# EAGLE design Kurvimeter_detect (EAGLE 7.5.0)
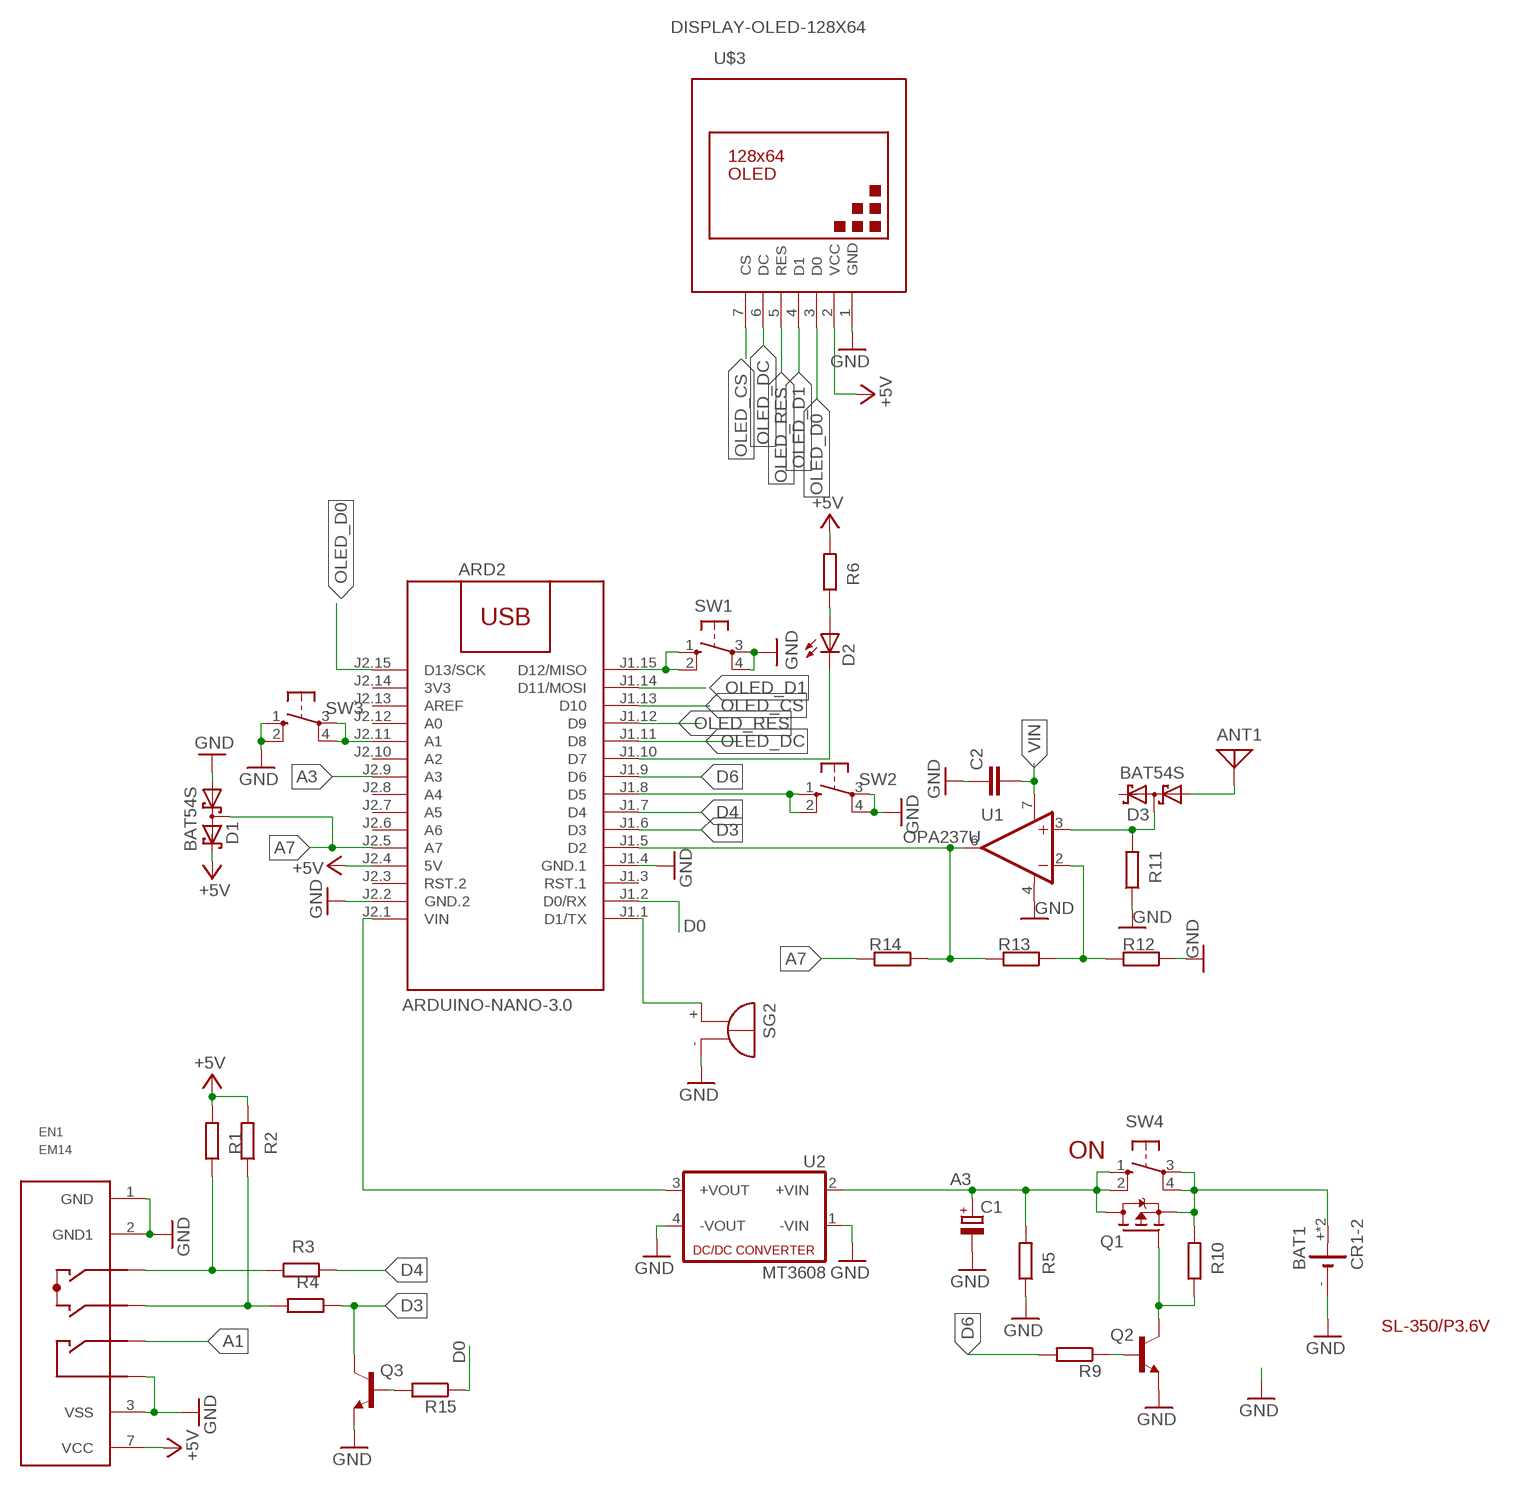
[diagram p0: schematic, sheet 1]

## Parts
ANT1  ANTENNA  [PAD-01]
ARD2  ARDUINO-NANO-3.0  [ARDUINO-NANO-3.0]
BAT1  CR1-2  [CR1-2]
C1  CPOL-EUSMCA  [SMC_A]
C2  C-EUC1206  [C1206]
D1  BAT54S  [SOT23]
D2  LED5MM  [LED5MM]
D3  BAT54S  [SOT23]
EN1  EM14  [EM14]
Q1  STR2P3LLH6  [SOT23]
Q2  BC817-16LT1SMD  [SOT23-BEC]
Q3  BC817-16LT1SMD  [SOT23-BEC]
R1  R-EU_R1206  [R1206]
R2  R-EU_R1206  [R1206]
R3  R-EU_R1206  [R1206]
R4  R-EU_R1206  [R1206]
R5  R-EU_R1206  [R1206]
R6  R-EU_R1206  [R1206]
R9  R-EU_R1206  [R1206]
R10  R-EU_R1206  [R1206]
R11  R-EU_R1206  [R1206]
R12  R-EU_R1206  [R1206]
R13  R-EU_R1206  [R1206]
R14  R-EU_R1206  [R1206]
R15  R-EU_R1206  [R1206]
SG2  BMT1205XH7.5  [BMT1205XH7.5]
SW1  10-XX  [B3F-10XX]
SW2  10-XX  [B3F-10XX]
SW3  10-XX  [B3F-10XX]
SW4  10-XX  [B3F-10XX]
U1  OPA237U  [SO08]
U2  MT3608  [MT3608]
U$3  DISPLAY-OLED-128X64  [DISPLAY-OLED-128X64]

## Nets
+5V: ARD2.J2.4(5V) D1.2(C2) EN1.7(VCC) R1.2 R2.2 R6.2 U$3.2(VCC)
A1: EN1.5(SW1)
A3: ARD2.J2.9(A3) C1.+ Q1.1(D) R5.2 SW4.1(S) SW4.2(S1) U2.2(+VIN)
A7: ARD2.J2.5(A7) D1.3(C1A2) R14.2
BAT: BAT1.+ BAT1.+@1(+) Q1.3(S) R10.2 SW4.3(P) SW4.4(P1)
D0: ARD2.J1.2(D0/RX) R15.1
D3: ARD2.J1.6(D3) Q3.C R4.1
D4: ARD2.J1.7(D4) R3.1
D6: ARD2.J1.9(D6) R9.2
GND: ARD2.J1.4(GND.1) ARD2.J2.2(GND.2) BAT1.- C1.- C2.1 D1.1(A1) EN1.1(GND) EN1.2(GND1) EN1.3(VSS) EN1.6(SW2) Q2.E Q3.E R5.1 R11.1 R12.1 SG2.- SW1.3(P) SW1.4(P1) SW2.3(P) SW2.4(P1) SW3.1(S) SW3.2(S1) U1.4(V-) U2.1(-VIN) U2.4(-VOUT) U$3.1(GND)
N$1: ARD2.J1.10(D7) D2.K(C)
N$2: ARD2.J1.8(D5) SW2.1(S) SW2.2(S1)
N$3: D3.3(C1A2) R11.2 U1.3(+IN)
N$4: D2.A R6.1
N$5: EN1.4(A) R1.1 R3.2
N$6: EN1.8(B) R2.1 R4.2
N$7: R12.2 R13.1 U1.2(-IN)
N$8: ARD2.J1.15(D12/MISO) SW1.1(S) SW1.2(S1)
N$9: ARD2.J1.5(D2) R13.2 R14.1 U1.6(OUT)
N$10: Q3.B R15.2
N$11: ANT1.1 D3.1(A1)
N$12: ARD2.J2.1(VIN) U2.3(+VOUT)
N$13: ARD2.J1.1(D1/TX) SG2.+
N$14: ARD2.J2.11(A1) SW3.3(P) SW3.4(P1)
N$16: Q1.2(G) Q2.C R10.1
N$18: Q2.B R9.1
OLED_CS: ARD2.J1.13(D10) U$3.7(CS)
OLED_D0: ARD2.J2.15(D13/SCK) U$3.3(D0)
OLED_D1: ARD2.J1.14(D11/MOSI) U$3.4(D1)
OLED_DC: ARD2.J1.11(D8) U$3.6(DC)
OLED_RES: ARD2.J1.12(D9) U$3.5(RES)
VIN: C2.2 U1.7(V+)
Unconnected: ARD2.J1.3(RST.1) ARD2.J2.3(RST.2) ARD2.J2.6(A6) ARD2.J2.7(A5) ARD2.J2.8(A4) ARD2.J2.10(A2) ARD2.J2.12(A0) ARD2.J2.13(AREF) D3.2(C2)

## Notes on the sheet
- ON
- SL-350/P3.6V

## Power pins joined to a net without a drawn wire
3V3: ARD2.J2.14(3V3)

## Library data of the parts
ANT1 = discrete:ANTENNA: Antenna
ARD2 = diy-modules:ARDUINO-NANO-3.0: Arduino Nano 3.0 and compatible devices More details available here: https://www.arduino.cc/en/Main/ArduinoBoardNano Click here to find device on ebay.com
BAT1 = battery:CR1-2
C1 = rcl:CPOL-EU: POLARIZED CAPACITOR, European symbol
C2 = rcl:C-EU: CAPACITOR, European symbol
D1 D3 = diode:BAT54S: Schottky Diodes Pin connection corrected 2011-05-04 Source: Fairchild .. BAT54.pdf
D2 = led:LED: LED
EN1 = switch-alps:EM14: 14 mm Rotary Optical Encoder w/Switch
Q1 = transistor-fet:STR2P3LLH6
Q2 Q3 = transistor-npn:BC817*: NPN Transistor
R1-R6 R9-R15 = rcl:R-EU_: RESISTOR, European symbol
SG2 = buzzer:BMT1205XH7.5: MAGNETIC TRANSDUCER; OC_FARNELL: unknown; OC_NEWARK: unknown
SW1-SW4 = switch-omron:10-XX: OMRON SWITCH; MPN: B3F-1000; OC_FARNELL: 176432; OC_NEWARK: 36M3542
U1 = burr-brown:OPA237: Operational Amplifiers Single-Supply, MicroAmplifier(TM) Series; MF: TEXAS INSTRUMENT CONNECTORS; MPN: OPA237UA; OC_FARNELL: 1800507; OC_NEWARK: 04M4584
U2 = dc-dc-converter:MT3608: DC DC Up Converter
U$3 = diy-modules:DISPLAY-OLED-128X64: 128x64 Dot Matrix OLED Module based on SSD1306 chip Variant with SPI interface More details available here: http://www.instructables.com/id/How-to-use-OLED-display-arduino-module/ SSD1306 datasheet: https://cdn-shop.adafruit.com/datasheets/SSD1306.pdf Click here to find device on ebay.com Note: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

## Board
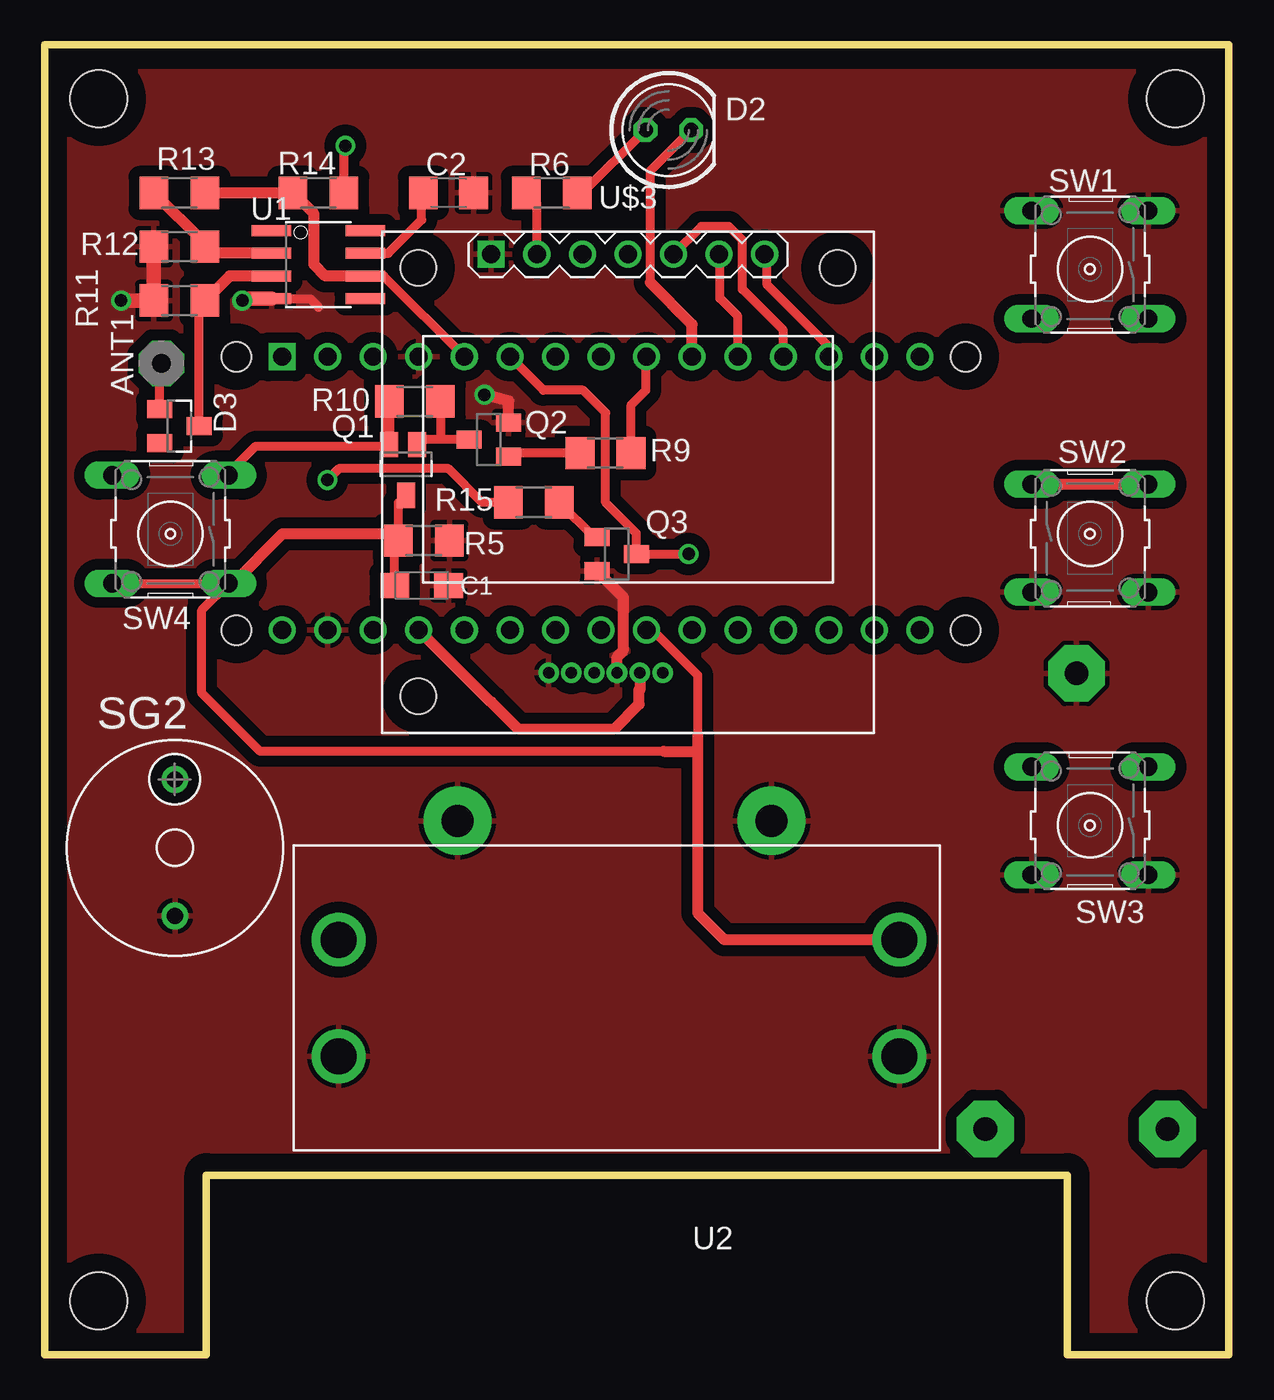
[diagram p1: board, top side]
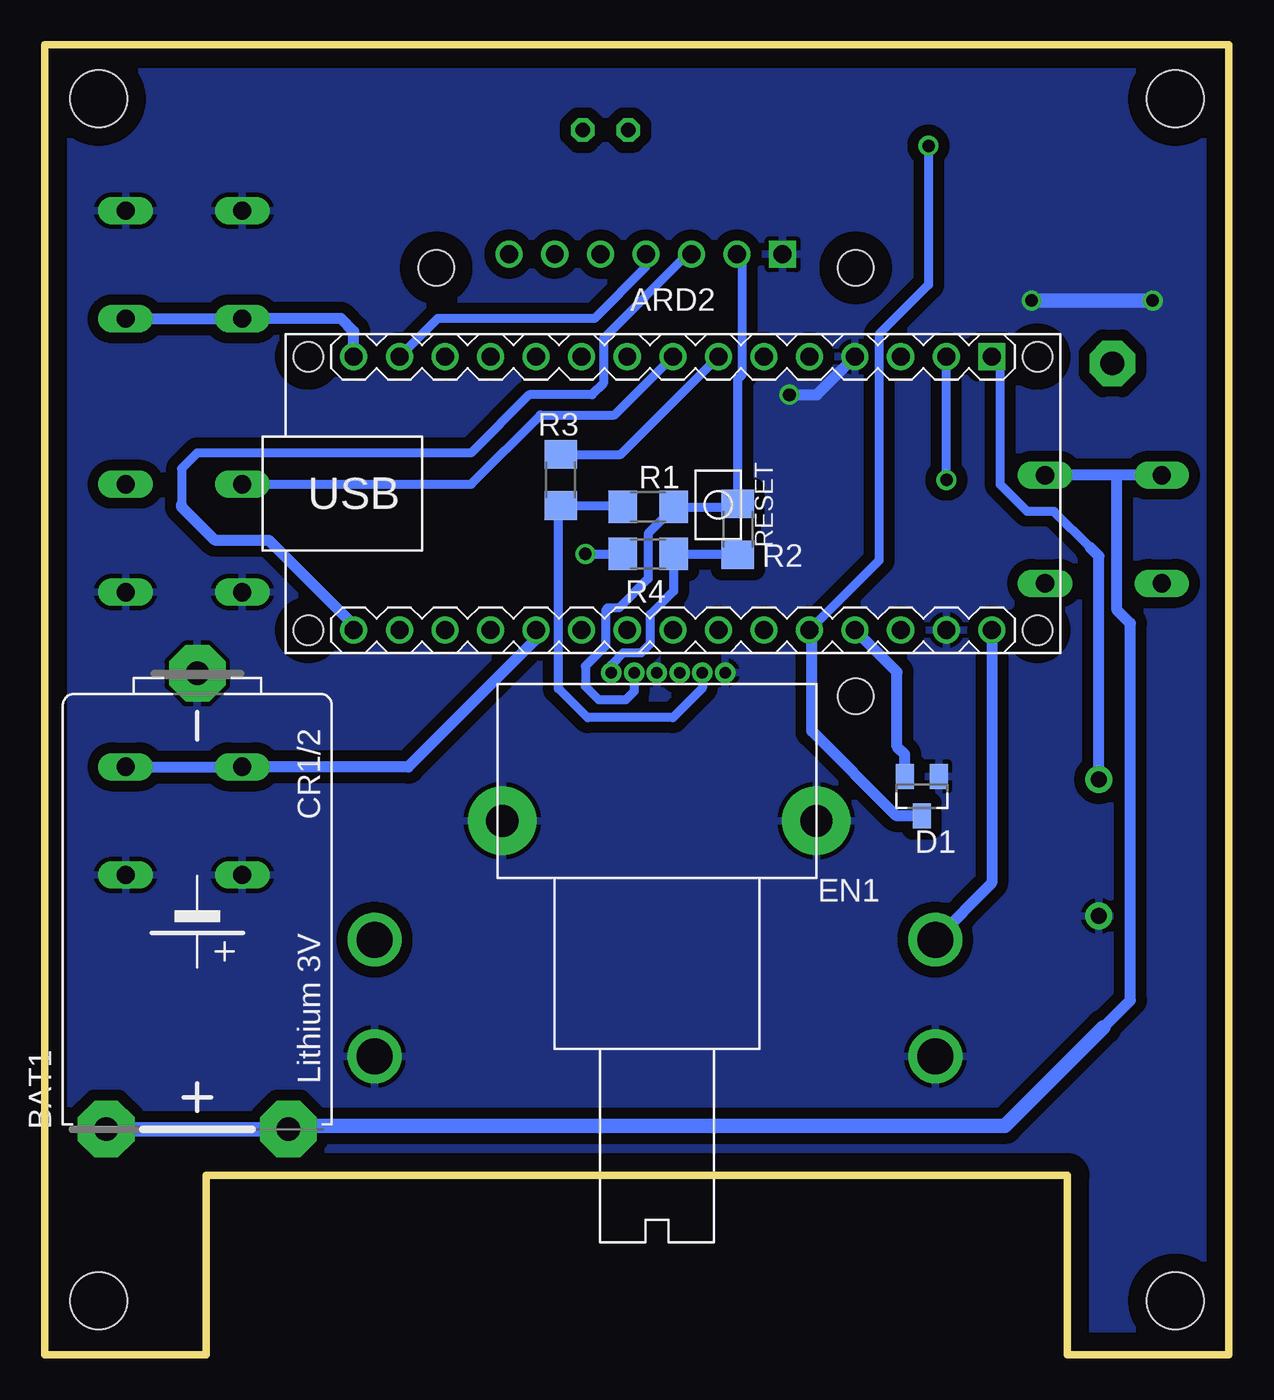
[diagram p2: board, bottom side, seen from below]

Size 66 x 73 mm. Coordinates in mm from the lower left corner, seen from the top.
Outline: 0,0 0,73 66,73 66,0 57,0 57,10 9,10 9,0 0,0
Copper layers (1*16): Top 0.035mm / dielectric 1.5mm / Bottom 0.035mm
Design rules "default *": minimum track width 10mil, minimum drill 15mil, track to track 6mil, track to pad 6mil, pad to pad 6mil, via to via 6mil, smd to smd 4mil, copper to edge 40mil, drill to drill 8mil, minimum pad ring 10mil, minimum via ring 8mil, stop-mask expansion 4mil, vias tented up to drill 0mil, thermal gap 10mil
Holes 3.2 mm at 3,70 63,70 3,3 63,3

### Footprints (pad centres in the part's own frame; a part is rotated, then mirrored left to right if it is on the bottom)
PAD-01 = drill 1.321 pad 2.54 octagon: 1 0,0
ARDUINO-NANO-3.0 = drill 1 square: J1.1 17.78,7.62 | drill 1: J1.2 15.24,7.62; J1.3 12.7,7.62; J1.4 10.16,7.62; J1.5 7.62,7.62; J1.6 5.08,7.62; J1.7 2.54,7.62; J1.8 0,7.62; J1.9 -2.54,7.62; J1.10 -5.08,7.62; J1.11 -7.62,7.62; J1.12 -10.16,7.62; J1.13 -12.7,7.62; J1.14 -15.24,7.62; J1.15 -17.78,7.62; J2.1 17.78,-7.62; J2.2 15.24,-7.62; J2.3 12.7,-7.62; J2.4 10.16,-7.62; J2.5 7.62,-7.62; J2.6 5.08,-7.62; J2.7 2.54,-7.62; J2.8 0,-7.62; J2.9 -2.54,-7.62; J2.10 -5.08,-7.62; J2.11 -7.62,-7.62; J2.12 -10.16,-7.62; J2.13 -12.7,-7.62; J2.14 -15.24,-7.62; J2.15 -17.78,-7.62 | hole 1.651: -20.32,7.62; -20.32,-7.62; 20.32,-7.62; 20.32,7.62
CR1-2 = drill 1.321 pad 3.15 octagon: + -11.43,-5.08; +@1 -11.43,5.08; - 13.97,0
SMC_A = smd 1.6 x 1.4: + -1.5,0; - 1.5,0
C1206 = smd 1.6 x 1.8: 1 -1.4,0; 2 1.4,0
SOT23 = smd 1 x 1.4: 1 -0.95,-1.1; 2 0.95,-1.1; 3 0,1.1
LED5MM = drill 0.813 octagon: A -1.27,0; K 1.27,0
EM14 = drill 1.8 pad 3.81: 1 0,0; 2 17.5,0 | drill 0.635 pad 0.889: 3 5.08,-8.255; 4 6.35,-8.255; 5 7.62,-8.255; 6 8.89,-8.255; 7 10.16,-8.255; 8 11.43,-8.255
SOT23' = smd 1 x 1.4: 1 0,1.735; 2 -0.632,-1.1; 3 0.95,-1.1
SOT23-BEC = smd 1 x 1.4: B -0.95,-1.1; C 0,1.1; E 0.95,-1.1
R1206 = smd 1.6 x 1.803: 1 -1.422,0; 2 1.422,0
BMT1205XH7.5 = drill 0.9 pad 1.5: + 3.8,0; - -3.8,0
B3F-10XX = drill 1.016 long: 1 -3.251,2.761; 2 3.251,2.761; 3 -3.251,-3.261; 4 3.251,-3.261
SO08 = smd 0.61 x 2.21: 1 -1.905,-2.616; 2 -0.635,-2.616; 3 0.635,-2.616; 4 1.905,-2.616; 5 1.905,2.616; 6 0.635,2.616; 7 -0.635,2.616; 8 -1.905,2.616
MT3608 = drill 2: 1 2.25,11.75; 2 2.25,5.25; 3 33.5,5.25; 4 33.5,11.75
DISPLAY-OLED-128X64 = drill 1 square: 1 -7.62,12.7 | drill 1: 2 -5.08,12.7; 3 -2.54,12.7; 4 0,12.7; 5 2.54,12.7; 6 5.08,12.7; 7 7.62,12.7 | hole 2: -11.684,11.938; 11.684,11.938; -11.684,-11.938

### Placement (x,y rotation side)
ANT1  6.5,55.25 0 top
ARD2  31,48 0 bottom
BAT1  57.5,24 90 bottom
C1  21,42.88 0 top
C2  22.5,64.75 180 top
D1  17.12,31.12 180 bottom
D2  34.75,68.25 0 top
D3  7.5,51.75 270 top
EN1  23,29.75 180 bottom
Q1  STR2P3LLH6  [SOT23']  20.12,49.62 180 top
Q2  24.75,51 90 top
Q3  31.88,44.62 270 top
R1  32.38,47.25 0 bottom
R2  27.38,46 90 bottom
R3  37.25,48.75 270 bottom
R4  32.38,44.62 0 bottom
R5  21.12,45.38 180 top
R6  28.25,64.75 180 top
R9  31.25,50.25 0 top
R10  20.62,53.12 180 top
R11  7.5,58.75 0 top
R12  7.5,61.75 0 top
R13  7.5,64.75 0 top
R14  15.25,64.75 0 top
R15  27.25,47.5 0 top
SG2  7.25,28.25 90 top
SW1  58.25,60.5 180 top
SW2  58.25,45.75 0 top
SW3  58.25,29.5 180 top
SW4  7,45.75 180 top
U1  15.25,60.75 270 top
U2  49.88,28.38 180 top
U$3  32.5,48.62 0 top

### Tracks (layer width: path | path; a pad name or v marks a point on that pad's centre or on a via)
+5V
  Top 0.5: U$3.2 27.42,64.16 R6.2
  Top 0.61: EN1.7 33.16,37.12 | 33.16,37.12 33.16,37.03 | ARD2.J2.4 24.84,36.38 24.88,36.38 26.38,34.88 31.75,34.88 33.12,36.25 33.12,37.09 33.16,37.12
  Bottom 0.5: U$3.2 27.12,61.03 27.12,54.62 27.38,54.38 R2.2 27.55,47.25 R1.2 30.95,47.17 32.38,45.75 32.38,43.25 34,41.62 34.62,41.62 34.75,41.5 34.75,39.5 35.88,38.38 35.88,37.25 35.12,36.5 33.62,36.5 33.16,36.97 EN1.7
  Bottom 0.61: D1.2 18.07,33.45 18.5,33.88 18.5,38.04 ARD2.J2.4
A3
  Top 0.5: C1.+ 19.5,45.17 R5.2 19.7,47.47 Q1.1 | ARD2.J2.9 33.87,40.38 36.38,37.88 36.38,34.5 | 34.5,33.62 12,33.62 8.75,36.88 8.75,41.49 SW4.1 SW4.2
  Top 0.61: SW4.1 10.49,42.99 13.25,45.75 19.33,45.75 R5.2 | U2.2 37.88,23.12 36.38,24.62 36.38,33.5 | 36.38,34.5 36.38,33.5 | 34.5,33.62 36.25,33.62 36.38,33.5
A7  (via drill 0.7)
  Top 0.5: R14.2 16.67,67.3 v16.75,67.38
  Bottom 0.5: v16.75,67.38 16.75,59.62 19.5,56.88 19.5,44.26 ARD2.J2.5
  Bottom 0.61: D1.3 18.52,30.02 23.25,34.75 23.25,40.25 ARD2.J2.5
BAT
  Top 0.5: SW4.3 10.25,49.13 11.75,50.62 19.07,50.62 Q1.3
  Top 0.61: Q1.3 19.18,53.1 R10.2
  Bottom 0.61: SW4.4 6.25,49.01 | 6.25,49.01 SW4.3 | 7,18.25 5.5,19.75 5.5,40.75 6.25,41.5 6.25,49.01
  Bottom 0.813: BAT1.+@1 BAT1.+ 52.24,12.75 12.5,12.75 7,18.25
D0  (via drill 0.7)
  Top 0.5: R15.1 24.38,47.5 22.5,49.38 16.38,49.38 v15.75,48.75
  Bottom 0.5: v15.75,48.75 ARD2.J1.2
D3  (via drill 0.7)
  Top 0.5: v35.88,44.62 Q3.C 32.98,45.77 31.25,47.5 31.25,52.5 30,53.75 27.79,53.75 ARD2.J1.6
  Bottom 0.5: v35.88,44.62 R4.1
D4
  Bottom 0.5: R3.1 33.91,50.17 ARD2.J1.7
D6
  Top 0.5: ARD2.J1.9 33.5,55.58 33.5,53.75 32.67,52.92 R9.2
GND  (via drill 0.7)
  Top 0.5: U1.4 14.78,58.84 15.25,58.38
  Top 0.61: R11.1 R12.1 | Q2.E 25.85,53.15 v24.5,53.5 | EN1.6 31.89,38.89 32.25,39.25 32.25,42.2 Q3.E
  Top 0.813: 6,61.62 6.08,61.55 R11.1 v4.25,58.75 | U1.4 11.1,58.84 v11,58.75
  Bottom 0.61: v24.5,53.5 22.96,53.5 ARD2.J1.4
  Bottom 0.813: v11,58.75 v4.25,58.75
  pour Top (isolate 0.61): 0.75,71.5 65.5,71.5 65.5,0.5 0.75,0
  pour Bottom (isolate 0.61): 1,71.5 65.38,71.5 65.38,0.75 1,0.75
N$1
  Top 0.5: 33.75,59.75 33.75,65.98 D2.K
  Top 0.61: ARD2.J1.10 36.08,57.42 33.75,59.75
N$2
  Top 0.61: SW2.1 SW2.2
  Bottom 0.5: SW2.1 42.24,48.51 38.38,52.38 34.24,52.38 ARD2.J1.8
N$3
  Top 0.5: D3.3 8.6,58.43 R11.2
  Top 0.61: U1.3 10.29,60.12 R11.2
N$4
  Top 0.5: R6.1 29.98,64.75 D2.A
N$5
  Bottom 0.5: EN1.4 29.35,37.15 31,35.5 35.75,35.5 37.38,37.12 37.38,47.2 R3.2 33.88,47.33 R1.1
N$6
  Bottom 0.5: R2.1 27.42,44.62 R4.2 30.95,42.55 32.25,41.25 32.25,39.62 32.75,39.12 33.75,39.12 34.43,38.45 EN1.8
N$7
  Top 0.61: R13.1 8.92,61.91 R12.2 9.29,61.38 U1.2
N$8
  Bottom 0.61: SW1.1 55.5,57.74 | 55.5,57.74 SW1.2 | ARD2.J1.15 48.78,57.03 49.5,57.75 55.49,57.75 55.5,57.74
N$9
  Top 0.5: U1.6 18.89,60.12 ARD2.J1.5
  Top 0.61: R13.2 R14.1 15,63.58 15,60.75 15.63,60.12 U1.6
N$10
  Top 0.5: Q3.B 30.6,45.58 R15.2
N$11
  Top 0.5: D3.1 6.4,55.15 ANT1.1
N$12
  Bottom 0.61: ARD2.J2.1 13.22,26.28 U2.3
N$13
  Bottom 0.5: 7.75,45 9.75,47 11.25,47 12.75,48.5 12.75,55.15 ARD2.J1.1
  Bottom 0.61: SG2.+ 7.25,44.5 7.75,45
N$14
  Bottom 0.61: SW3.3 SW3.4 54.99,32.75 45.75,32.75 38.62,39.88 ARD2.J2.11
N$16
  Top 0.5: Q2.C 22,51 | 22,51 21.03,51 Q1.2 | R10.1 22.05,51.05 22,51
N$18
  Top 0.5: R9.1 26.05,50.25 Q2.B
OLED_CS
  Top 0.5: ARD2.J1.13 43.7,56.17 40.25,59.62 40.25,61.2 U$3.7
OLED_D0
  Bottom 0.5: U$3.3 30.18,61.33 34.88,56.62 34.88,54.12 35.5,53.5 39,53.5 42.25,50.25 57.5,50.25 58.38,49.38 58.38,47.38
  Bottom 0.61: ARD2.J2.15 48.78,40.66 53.5,45.38 56.5,45.38 58.38,47.25 58.38,47.38
OLED_D1
  Bottom 0.5: U$3.4 32.5,60.62 35.38,57.75 44.11,57.75 ARD2.J1.14
OLED_DC
  Top 0.5: ARD2.J1.11 38.62,57.88 37.62,58.88 37.62,61.28 U$3.6
OLED_RES
  Top 0.5: ARD2.J1.12 41.16,57.09 38.88,59.38 38.88,62.12 38.12,62.88 36.59,62.88 U$3.5
VIN
  Top 0.5: U1.7 19.14,61.38 21,63.25 21,64.65 C2.2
